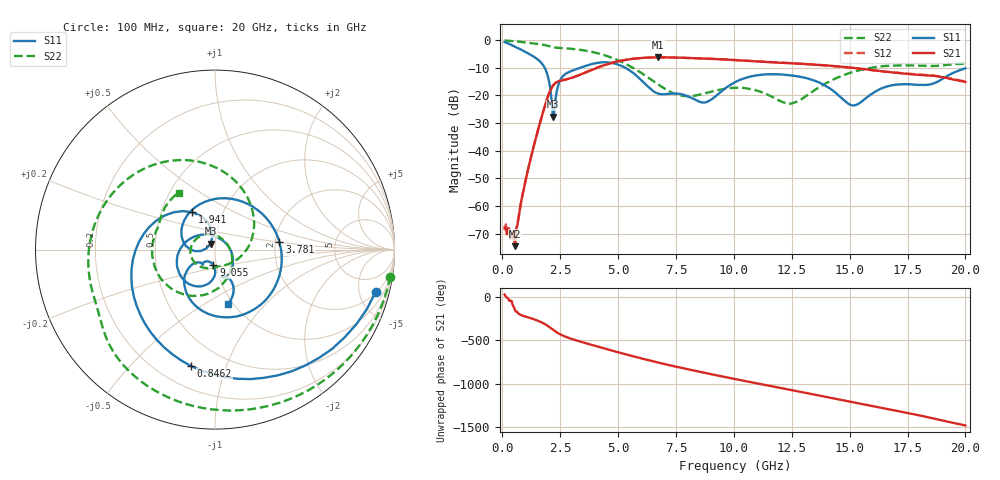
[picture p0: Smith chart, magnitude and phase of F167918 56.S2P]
!  2-Port S-parameters saved by WinCal
! VAR MeasName=S-Parameters (CALIBRATED_DATA) read from VNA (N5242A)
! VAR MeasDate=2016-11-22 10:27:33
! VAR NAME=F167918 56
! VAR FILENAME=F167918 56.S2P
! VAR DATE=2016-11-22 10:27:33
! VAR PHYS_PORTS=1,2
# Hz S DB R 50
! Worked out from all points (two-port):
!   401 points, 100 MHz to 20 GHz, reference 50 ohm
!   highest |S21| = -6.20 dB at 6.717 GHz (marker M1); lowest = -74.5 dB at 547.8 MHz (marker M2)
!   |S21| within 3 dB of the highest: 4.346 GHz to 14.11 GHz (9.762 GHz wide, 106 % of centre)
!   lowest |S11| = -27.7 dB at 2.189 GHz (marker M3), VSWR 1.09, Z = 47.5 + j3.2 ohm
!   |S11| at or under -10 dB: 1.832 GHz to 3.358 GHz (1.526 GHz wide, 58.8 % of centre); 5.316 GHz to end of sweep
!   |S22| runs from -23.0 to -0.1 dB; largest |S21 - S12| = 0.0042
!   S11 on the Smith chart (normalised r, x): 100 MHz: 2.13, -7.07; 846.2 MHz: 0.33, -0.76; 1.941 GHz: 0.72, +0.32; 3.781 GHz: 2.11, +0.20; 9.055 GHz: 0.97, -0.17; 20 GHz: 0.95, -0.64
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1e8  -0.67 -14.8  -67.79 30.5  -68.79 33.7  -0.10 -8.7
5.4775e8  -2.33 -69.0  -74.50 -148.6  -74.23 -160.0  -0.40 -44.8
8.4625e8  -3.58 -101.6  -57.02 149.8  -56.94 148.5  -0.67 -67.2
1.3935e9  -6.15 -161.1  -37.16 102.4  -37.12 102.5  -1.21 -104.0
1.94075e9  -12.25 121.5  -21.11 32.2  -21.09 32.3  -1.97 -136.7
2.1895e9  -27.65 125.7  -16.44 -16.3  -16.43 -16.1  -2.53 -148.7
2.5875e9  -13.32 150.1  -14.53 -80.8  -14.49 -80.8  -2.87 -165.3
3.43325e9  -9.78 42.8  -12.24 -158.5  -12.24 -158.5  -3.58 156.5
3.7815e9  -8.84 6.4  -11.03 174.6  -11.02 174.7  -4.08 140.5
4.52775e9  -8.02 -60.1  -8.72 118.2  -8.69 118.2  -5.75 105.5
5.1745e9  -9.41 -106.1  -7.36 70.5  -7.33 70.4  -7.94 74.2
6.71675e9  -19.28 -138.0  -6.20 -35.1  -6.21 -35.1  -15.94 -8.2
6.7665e9  -19.41 -136.8  -6.21 -38.2  -6.21 -38.3  -16.21 -11.3
7.81125e9  -19.71 -131.2  -6.37 -101.7  -6.36 -101.5  -20.14 -69.2
9.055e9  -21.31 -95.9  -6.74 -172.1  -6.73 -172.1  -18.59 -120.8
1.005e10  -15.20 -96.0  -7.18 133.4  -7.17 133.6  -17.23 -162.1
1.199025e10  -12.37 -143.3  -8.16 31.9  -8.09 31.6  -22.01 88.2
1.338325e10  -14.38 177.6  -8.77 -41.5  -8.77 -41.7  -18.69 -34.2
1.51245e10  -23.61 59.1  -9.99 -134.2  -10.03 -134.3  -11.54 -105.8
1.67165e10  -16.56 -55.8  -11.51 142.1  -11.54 142.5  -9.25 -156.2
1.875625e10  -15.18 -64.8  -13.04 30.0  -12.94 30.3  -9.27 154.5
2e10  -10.16 -76.1  -15.10 -43.0  -14.95 -43.0  -8.50 122.7
